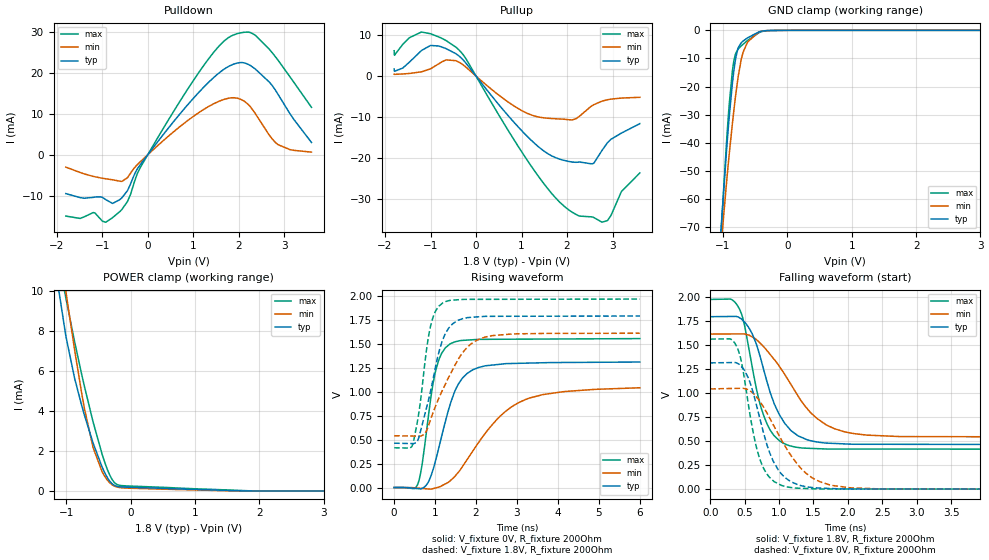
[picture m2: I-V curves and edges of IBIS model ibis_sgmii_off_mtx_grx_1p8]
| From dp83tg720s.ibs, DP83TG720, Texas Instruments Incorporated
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|   ibis_sgmii_off_mtx_grx_1p8
[Model]   ibis_sgmii_off_mtx_grx_1p8
Model_type   I/O
Polarity   Non-Inverting
Enable   Active-Low
Vinl = 0.54
Vinh = 1.26
Vmeas = 0.9
Vref = 0
Cref = 2pF
Rref = 100000
|   typ   min   max
C_comp   3.49pF   3.38pF   3.6pF
[Voltage Range]   1.8   1.62   1.98
[Temperature Range]   27   150   -40
[Pullup Reference]   1.8   1.62   1.98
[Pulldown Reference]   -0   0   0
[Power Clamp Reference]   1.8   1.62   1.98
[GND Clamp Reference]   0   0   0
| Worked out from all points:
|   slope of the pulldown table from 0 to 0.27 V, typ, clamps not added: 68.8 ohm
|   slope of the pullup table from 0 to 0.27 V, typ, clamps not added: 71.1 ohm
|   GND clamp passes 1 mA (typ) near -0.48 V on its own axis
|   POWER clamp passes 1 mA (typ) near -0.42 V on its own axis
|   falling waveform, V_fixture 1.8V, R_fixture 200Ohm: 20-80 % time 383ps typ, 646ps min, 288ps max; typ from 1.79 V to 0.463 V
|   rising waveform, V_fixture 0V, R_fixture 200Ohm: 20-80 % time 530ps typ, 1.18ns min, 325ps max; typ from 0 V to 1.31 V
|   rising waveform, V_fixture 1.8V, R_fixture 200Ohm: 20-80 % time 443ps typ, 728ps min, 292ps max; typ from 0.463 V to 1.79 V
|   falling waveform, V_fixture 0V, R_fixture 200Ohm: 20-80 % time 334ps typ, 537ps min, 248ps max; typ from 1.31 V to 0 V
[Pulldown]
|   Voltage   I(typ)   I(min)   I(max)
-1.8V     -9.479mA   -3.004mA   -14.98mA
-1.195V   -10.4mA    -5.276mA   -14.1mA
-925.2mV  -10.92mA   -5.852mA   -16.47mA
-568.8mV  -10.52mA   -6.501mA   -13.38mA
-444.6mV  -8.758mA   -5.595mA   -11.42mA
-153mV    -2.253mA   -1.597mA   -2.917mA
765mV     10.75mA    7.393mA    14.08mA
1.445V    18.84mA    12.45mA    24.98mA
1.872V    22.09mA    13.95mA    29.24mA
2.363V    20.99mA    10.11mA    29.25mA
2.866V    14.76mA    2.481mA    23.12mA
3.6V      3.022mA    656.1uA    11.6mA
[GND Clamp]
|   Voltage   I(typ)   I(min)   I(max)
-1.8V     -377.4mA   -335mA     -413.9mA
-1.033V   -71.68mA   -77.46mA   -72.71mA
-1.022V   -67.89mA   -74.41mA   -68.39mA
-941.4mV  -41.35mA   -53.02mA   -38.15mA
-903.6mV  -30.6mA    -43.97mA   -26.23mA
-833.4mV  -14.6mA    -28.74mA   -11.04mA
-768.6mV  -6.515mA   -17.05mA   -6.746mA
-720mV    -4.478mA   -10.63mA   -5.603mA
-617.4mV  -2.643mA   -4.104mA   -3.572mA
-444.6mV  -591.6uA   -614.2uA   -888uA
-309.6mV  -92.11uA   -92.87uA   -124.5uA
3.6V      0A         0A         0A
[Pullup]
|   Voltage   I(typ)   I(min)   I(max)
-1.8V     1.744mA    480.8uA    6.165mA
-1.206V   6.14mA     1.032mA    10.69mA
-828mV    7.327mA    2.927mA    9.562mA
-444.6mV  5.46mA     3.759mA    7.052mA
716.4mV   -9.749mA   -6.381mA   -13.38mA
1.316V    -16.64mA   -9.796mA   -23.51mA
1.823V    -20.13mA   -10.42mA   -30.47mA
2.25V     -20.92mA   -9.965mA   -33.92mA
2.59V     -21.16mA   -6.937mA   -34.39mA
2.882V    -16.3mA    -5.763mA   -35.15mA
3.195V    -13.86mA   -5.339mA   -28.08mA
3.6V      -11.56mA   -5.156mA   -23.55mA
[POWER Clamp]
|   Voltage   I(typ)   I(min)   I(max)
-1.8V     53.03mA    32.09mA    32.8mA
-1.13V    10.31mA    12.75mA    11.79mA
-1.006V   7.723mA    9.944mA    9.63mA
-871.2mV  5.628mA    7.042mA    7.462mA
-720mV    3.797mA    4.133mA    5.24mA
-585mV    2.398mA    2.165mA    3.454mA
-444.6mV  1.193mA    960.8uA    1.835mA
-347.4mV  586.3uA    482.8uA    949uA
-271.8mV  317uA      273uA      491.5uA
-142.2mV  198.3uA    155.7uA    266.6uA
1.067V    69.48uA    43.47uA    98.18uA
3.6V      0A         0A         0A
[Ramp]
R_load = 200
|   typ   min   max
dV/dt_r   0.785344/5.2842e-10   0.624336/1.18312e-09   0.931839/3.22318e-10
dV/dt_f   0.796488/3.80535e-10   0.641765/6.41741e-10   0.932979/2.87172e-10
[Falling Waveform]
V_fixture = 1.8V
V_fixture_min = 1.62V
V_fixture_max = 1.98V
R_fixture = 200Ohm
C_fixture = 0F
|   Time   V(typ)   V(min)   V(max)
0s        1.791V     1.61V      1.97V
420.1ps   1.782V     1.612V     1.877V
498ps     1.734V     1.611V     1.704V
609ps     1.615V     1.581V     1.275V
774ps     1.25V      1.481V     772.2mV
931.9ps   884.6mV    1.345V     553.3mV
1.126ns   648.3mV    1.143V     457.7mV
1.554ns   489.6mV    732.9mV    420.9mV
2.103ns   466.4mV    575.4mV    416.7mV
6ns       463mV      540.8mV    415mV
[Rising Waveform]
V_fixture = 0V
V_fixture_min = 0V
V_fixture_max = 0V
R_fixture = 200Ohm
C_fixture = 0F
|   Time   V(typ)   V(min)   V(max)
0s        289.8uV    154.2uV    462uV
570.2ps   -10.93mV   -5.183mV   28.71mV
679.8ps   -8.253mV   -9.085mV   233.9mV
818.7ps   45.43mV    -14.02mV   682.6mV
1.003ns   267.5mV    -5.325mV   1.198V
1.362ns   857.6mV    68.36mV    1.497V
1.578ns   1.086V     164.5mV    1.529V
1.919ns   1.228V     380.1mV    1.542V
3.007ns   1.295V     878.4mV    1.548V
6ns       1.309V     1.041V     1.554V
[Rising Waveform]
V_fixture = 1.8V
V_fixture_min = 1.62V
V_fixture_max = 1.98V
R_fixture = 200Ohm
C_fixture = 0F
|   Time   V(typ)   V(min)   V(max)
0s        462.8mV    540.4mV    414.9mV
457.6ps   458.5mV    537.2mV    452.9mV
590.9ps   505.8mV    536.3mV    746.4mV
872.9ps   974.6mV    688mV      1.652V
1.003ns   1.242V     840.7mV    1.832V
1.187ns   1.541V     1.021V     1.926V
1.424ns   1.707V     1.227V     1.955V
1.702ns   1.764V     1.423V     1.963V
2.24ns    1.786V     1.571V     1.963V
6ns       1.789V     1.609V     1.966V
[Falling Waveform]
|Gnd
V_fixture = 0V
V_fixture_min = 0V
V_fixture_max = 0V
R_fixture = 200Ohm
C_fixture = 0F
|   Time   V(typ)   V(min)   V(max)
0s        1.311V     1.041V     1.558V
384.1ps   1.311V     1.047V     1.484V
457.6ps   1.269V     1.048V     1.309V
553ps     1.156V     1.03V      888.5mV
710ps     767mV      924.8mV    337.8mV
865.3ps   376.9mV    736.5mV    121.3mV
1.033ns   160.1mV    515.3mV    39.95mV
1.386ns   26.52mV    168.6mV    7.256mV
1.767ns   6.786mV    39.59mV    2.118mV
6ns       498.9uV    154.2uV    547.4uV
